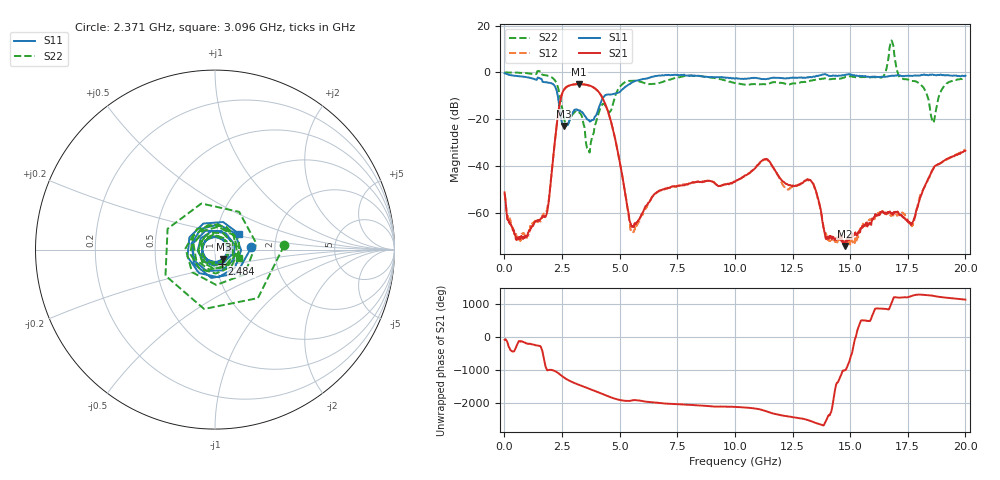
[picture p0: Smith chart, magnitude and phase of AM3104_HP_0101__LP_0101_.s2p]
!Created with skrf (http://scikit-rf.org).
# Hz S RI R 50.0
!freq ReS11 ImS11 ReS21 ImS21 ReS12 ImS12 ReS22 ImS22
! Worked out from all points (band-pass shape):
!   1601 points, 10 MHz to 20 GHz, reference 50 ohm
!   highest |S21| = -5.01 dB at 3.246 GHz (marker M1); lowest = -74.2 dB at 14.78 GHz (marker M2)
!   |S21| within 3 dB of the highest: 2.552 GHz to 4.059 GHz (1.508 GHz wide, 45.6 % of centre)
!   lowest |S11| = -22.9 dB at 2.584 GHz (marker M3), VSWR 1.15, Z = 54.6 - j5.94 ohm
!   |S11| at or under -10 dB: 2.316 GHz to 4.352 GHz (2.036 GHz wide, 61.1 % of centre)
!   |S22| runs from -34.3 to 13.6 dB; largest |S21 - S12| = 0.031
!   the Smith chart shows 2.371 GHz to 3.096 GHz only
!   S11 on the Smith chart (normalised r, x): 2.371 GHz: 1.51, +0.04; 2.484 GHz: 1.07, -0.17; 3.096 GHz: 1.29, +0.23
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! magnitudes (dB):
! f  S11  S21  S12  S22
! 10 MHz  -0.4  -51.3  -51.9  0.0
! 622.2 MHz  -1.7  -71.2  -71.8  -0.2
! 1.772 GHz  -4.2  -61.8  -60.2  -1.2
! 2.371 GHz  -13.9  -15.0  -15.1  -8.3
! 2.484 GHz  -21.0  -9.7  -9.8  -14.1
! 2.584 GHz  -22.9  -7.5  -7.5  -19.4
! 3.096 GHz  -15.9  -5.1  -5.1  -16.8
! 3.246 GHz  -16.4  -5.0  -5.1  -17.3
! 3.346 GHz  -16.9  -5.1  -5.2  -18.3
! 3.646 GHz  -20.3  -5.5  -5.6  -32.8
! 4.458 GHz  -9.5  -15.6  -15.6  -15.6
! 5.532 GHz  -4.3  -66.1  -67.9  -3.6
! 6.682 GHz  -1.4  -50.8  -50.9  -4.6
! 10.01 GHz  -2.7  -46.8  -46.7  -4.6
! 11.33 GHz  -2.9  -37.1  -37.3  -5.1
! 13.34 GHz  -2.1  -46.9  -47.1  -3.5
! 13.97 GHz  -1.0  -71.1  -69.3  -2.7
! 14.78 GHz  -1.1  -74.2  -73.3  -2.1
! 16.68 GHz  -1.6  -59.9  -60.8  7.2
! 17.69 GHz  -1.6  -64.6  -65.2  -3.7
! 18.59 GHz  -1.0  -41.5  -41.6  -21.1
! 20 GHz  -1.5  -33.5  -33.1  -2.5
